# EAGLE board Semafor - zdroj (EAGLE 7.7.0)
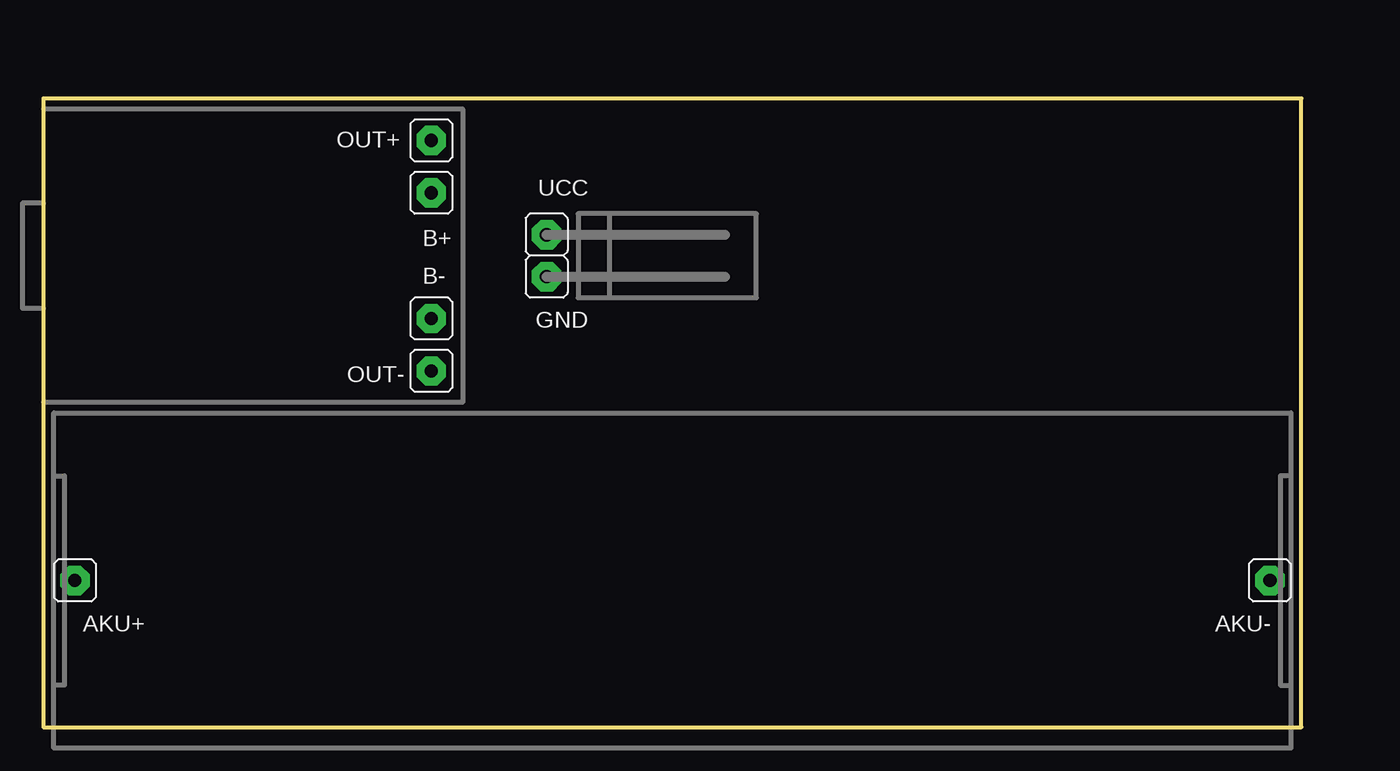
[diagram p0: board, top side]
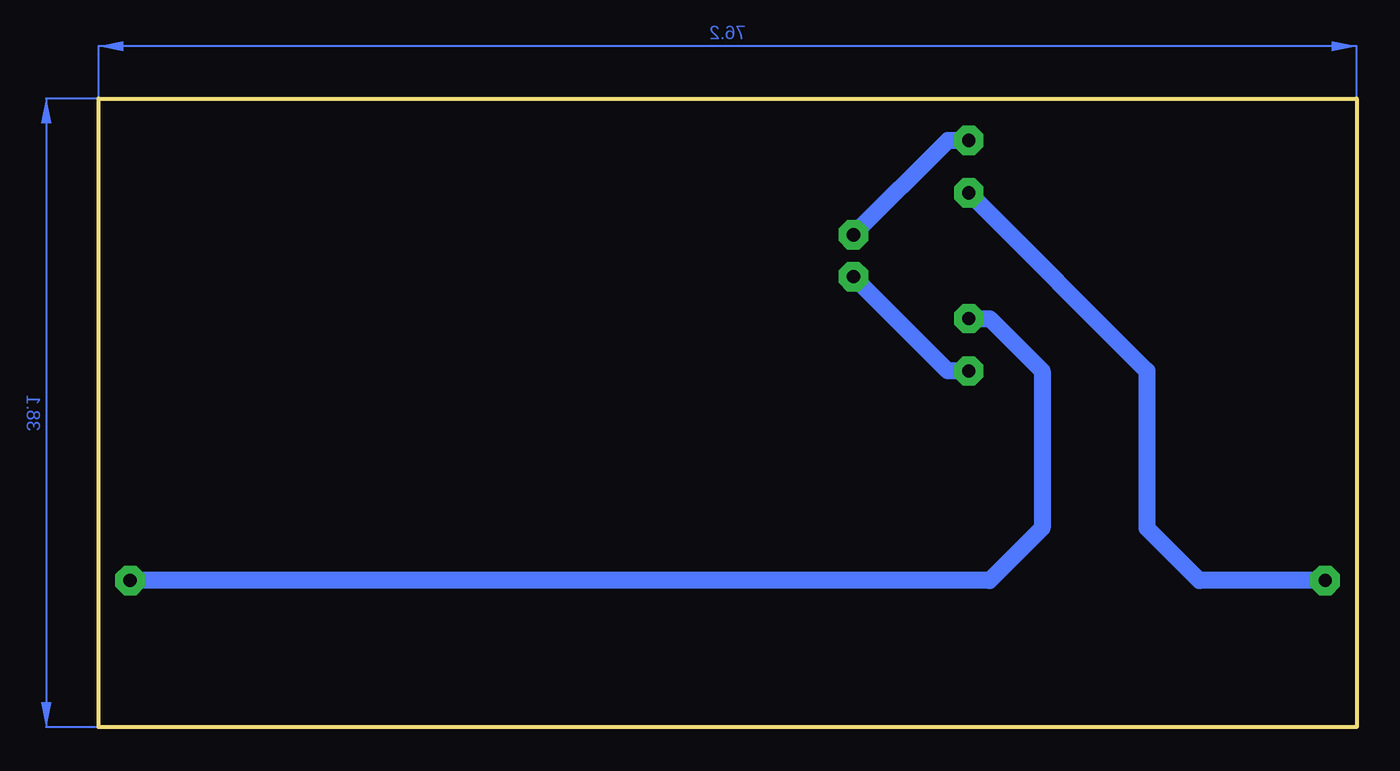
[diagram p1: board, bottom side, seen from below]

Size 76.2 x 38.1 mm. Coordinates in mm from the lower left corner, seen from the top.
Outline: 0,0 76.2,0 76.2,38.1 0,38.1 0,0
Copper layers (1*16): Top 0.035mm / dielectric 1.5mm / Bottom 0.035mm
Design rules "default": minimum track width 10mil, minimum drill 24mil, track to track 8mil, track to pad 8mil, pad to pad 8mil, via to via 8mil, smd to smd 8mil, copper to edge 40mil, drill to drill 8mil, minimum pad ring 10mil, minimum via ring 8mil, stop-mask expansion 4mil, vias tented up to drill 0mil, thermal gap 10mil

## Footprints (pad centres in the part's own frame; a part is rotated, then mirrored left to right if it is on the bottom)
S1G1_JUM = drill 0.8 pad 1.778 octagon: 1 0,0

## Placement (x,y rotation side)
AKU+  S1G1_JUMP  [S1G1_JUM]  1.91,8.89 0 top
AKU-  S1G1_JUMP  [S1G1_JUM]  74.3,8.89 0 top
B+  S1G1_JUMP  [S1G1_JUM]  23.5,32.38 0 top
B-  S1G1_JUMP  [S1G1_JUM]  23.5,24.77 0 top
GND  S1G1_JUMP  [S1G1_JUM]  30.48,27.3 0 top
OUT+  S1G1_JUMP  [S1G1_JUM]  23.5,35.56 0 top
OUT-  S1G1_JUMP  [S1G1_JUM]  23.5,21.59 0 top
UCC  S1G1_JUMP  [S1G1_JUM]  30.48,29.84 0 top

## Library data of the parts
AKU+ AKU- B+ B- GND OUT+ OUT- UCC = #PaJa_konektory

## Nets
N$1: AKU-.1 B-.1
N$2: OUT+.1 UCC.1
N$3: GND.1 OUT-.1
N$4: AKU+.1 B+.1

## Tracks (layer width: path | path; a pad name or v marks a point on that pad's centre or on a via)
N$1
  Bottom 1.016: AKU-.1 22.23,8.89 19.05,12.06 19.05,21.59 22.23,24.77 B-.1
N$2
  Bottom 1.016: OUT+.1 24.77,35.56 UCC.1
N$3
  Bottom 1.016: OUT-.1 24.77,21.59 GND.1
N$4
  Bottom 1.016: AKU+.1 9.53,8.89 12.7,12.06 12.7,21.59 B+.1
(copper drawn outside any net)
  shapes: Bottom area x2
